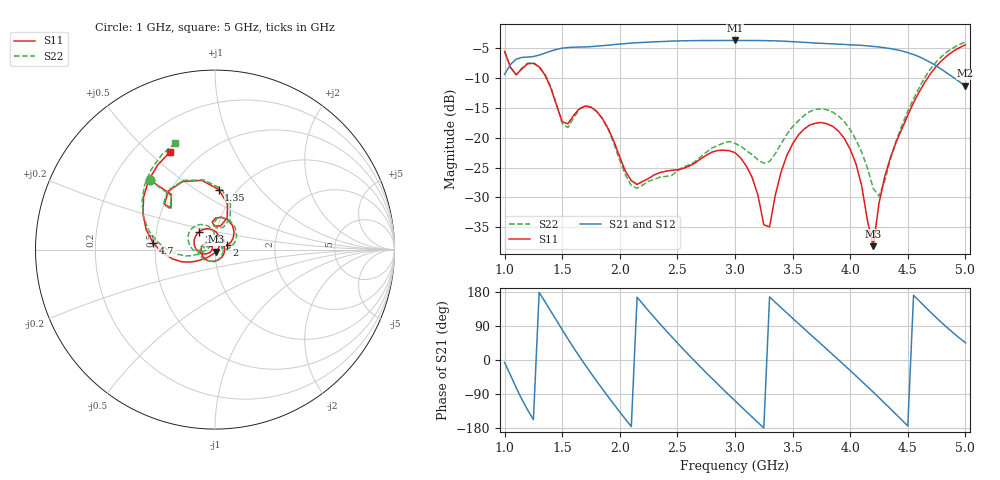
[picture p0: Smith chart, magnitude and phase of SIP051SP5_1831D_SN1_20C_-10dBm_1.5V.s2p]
# GHz  S  dB  R  50
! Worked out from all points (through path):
!   81 points, 1 GHz to 5 GHz, reference 50 ohm
!   highest |S21| = -3.70 dB at 3 GHz (marker M1); lowest = -11.3 dB at 5 GHz (marker M2)
!   lowest |S11| = -38.2 dB at 4.2 GHz (marker M3), VSWR 1.02, Z = 50.5 - j1.15 ohm
!   |S11| at or under -10 dB: 1.362 GHz to 4.672 GHz (3.31 GHz wide, 110 % of centre)
!   |S22| runs from -29.8 to -4.0 dB; largest |S21 - S12| = 0.0039
!   S11 on the Smith chart (normalised r, x): 1 GHz: 0.36, +0.39; 1.35 GHz: 0.83, +0.63; 2 GHz: 1.14, +0.05; 3.75 GHz: 0.82, +0.16; 4.7 GHz: 0.49, +0.04; 5 GHz: 0.34, +0.59
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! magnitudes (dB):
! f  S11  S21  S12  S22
! 1 GHz  -5.5  -9.4  -9.4  -5.5
! 1.1 GHz  -9.4  -6.8  -6.8  -9.5
! 1.35 GHz  -9.5  -5.8  -5.8  -9.3
! 1.5 GHz  -17.3  -5.0  -5.0  -17.6
! 1.7 GHz  -14.7  -4.8  -4.8  -14.7
! 1.85 GHz  -16.8  -4.6  -4.6  -16.8
! 2 GHz  -23.3  -4.3  -4.3  -23.8
! 2.15 GHz  -27.8  -4.1  -4.1  -28.5
! 2.35 GHz  -25.8  -3.9  -3.9  -26.6
! 3 GHz  -22.5  -3.7  -3.7  -21.0
! 3.15 GHz  -26.7  -3.7  -3.7  -22.9
! 3.25 GHz  -34.6  -3.7  -3.7  -24.3
! 3.3 GHz  -34.9  -3.7  -3.7  -24.0
! 3.45 GHz  -23.0  -3.8  -3.8  -19.4
! 3.7 GHz  -17.6  -4.1  -4.1  -15.2
! 3.75 GHz  -17.5  -4.2  -4.2  -15.1
! 4 GHz  -21.9  -4.4  -4.4  -18.7
! 4.2 GHz  -38.2  -4.7  -4.7  -28.5
! 4.25 GHz  -31.0  -4.8  -4.8  -29.8
! 4.35 GHz  -23.3  -5.1  -5.1  -23.5
! 4.7 GHz  -9.2  -7.4  -7.4  -8.4
! 5 GHz  -4.4  -11.3  -11.3  -4.0
